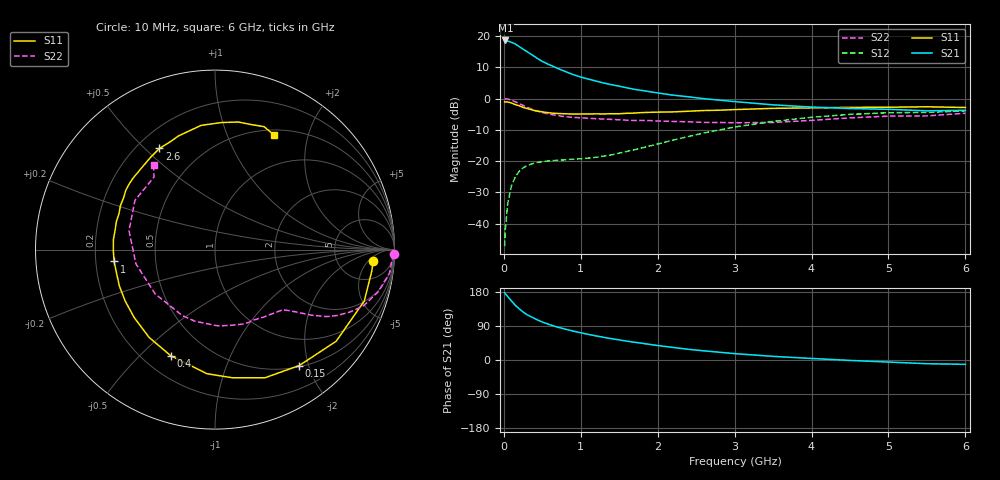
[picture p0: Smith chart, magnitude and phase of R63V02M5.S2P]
! SIEMENS Small Signal Semiconductors
! BFR193
! Si NPN RF Bipolar Junction Transistor in SOT23
! VCE = 3 V  IC = 2.5 mA
! Common Emitter S-Parameters:  May  1996
# GHz  S  MA  R  50
!  f  S11  S21  S12  S22
! GHz  MAG  ANG  MAG  ANG  MAG  ANG  MAG  ANG
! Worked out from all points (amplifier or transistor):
!   36 points, 10 MHz to 6 GHz, reference 50 ohm
!   highest |S21| = 18.5 dB at 20 MHz (marker M1)
!   |S21| within 3 dB of that: start of sweep to 265.2 MHz
!   unconditionally stable (mu >= 1): 1.103 GHz to 2.007 GHz
!   at 250 MHz: K = 0.27, MSG = 18.9 dB, |S12| = -22.1 dB
!   at 1.4 GHz: K = 1.10, MAG = 9.3 dB, |S12| = -18.0 dB
!   at 6 GHz: K = 0.99, MSG = 0.1 dB, |S12| = -3.9 dB
!   S11 on the Smith chart (normalised r, x): 10 MHz: 12, -7; 150 MHz: 0.52, -1.85; 400 MHz: 0.31, -0.62; 1 GHz: 0.28, -0.05; 2.6 GHz: 0.29, +0.55; 6 GHz: 0.56, +1.49
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0.01  0.8834 -4.0  8.304 177.8  0.0044 87.1  0.9958 -1.5
0.02  0.8817 -7.8  8.44 174.8  0.0083 85.3  0.989 -3.0
0.05  0.8796 -19.0  8.273 167.5  0.0211 79.9  0.9807 -7.7
0.1  0.8465 -37.1  7.88 155.7  0.0408 71.1  0.94 -14.4
0.15  0.7984 -54.0  7.404 144.0  0.0566 62.0  0.8859 -20.6
0.2  0.7665 -68.7  6.738 135.0  0.069 55.7  0.8303 -24.7
0.25  0.7206 -82.3  6.138 126.7  0.0782 50.4  0.776 -28.2
0.3  0.6929 -93.7  5.618 119.6  0.0848 46.7  0.7251 -31.0
0.4  0.6407 -112.6  4.66 109.4  0.0934 40.9  0.6484 -34.3
0.5  0.6117 -126.9  3.904 100.2  0.0984 37.6  0.5978 -36.3
0.6  0.5883 -139.9  3.422 92.9  0.1018 36.2  0.5611 -38.0
0.7  0.5767 -150.3  3.023 86.7  0.103 36.5  0.5332 -39.6
0.8  0.5699 -159.3  2.693 81.3  0.1052 37.2  0.5121 -41.1
1  0.5662 -173.3  2.202 71.8  0.109 40.5  0.4919 -44.6
1.1  0.5665 -179.8  2.04 67.5  0.1122 42.9  0.4837 -46.9
1.6  0.5812 155.0  1.48 49.7  0.143 55.7  0.4511 -59.5
2.2  0.6115 132.3  1.131 33.2  0.2171 61.4  0.4302 -79.4
2.6  0.6429 118.8  0.995 24.2  0.2813 59.1  0.4155 -96.3
3.5  0.6964 96.4  0.792 9.6  0.4305 44.7  0.4147 -143.3
4.5  0.7224 79.7  0.692 -1.1  0.5579 24.9  0.4906 167.6
5.5  0.7376 68.3  0.636 -9.8  0.5997 6.1  0.5281 130.1
6  0.7182 62.7  0.648 -11.4  0.6353 0.9  0.5818 126.0
